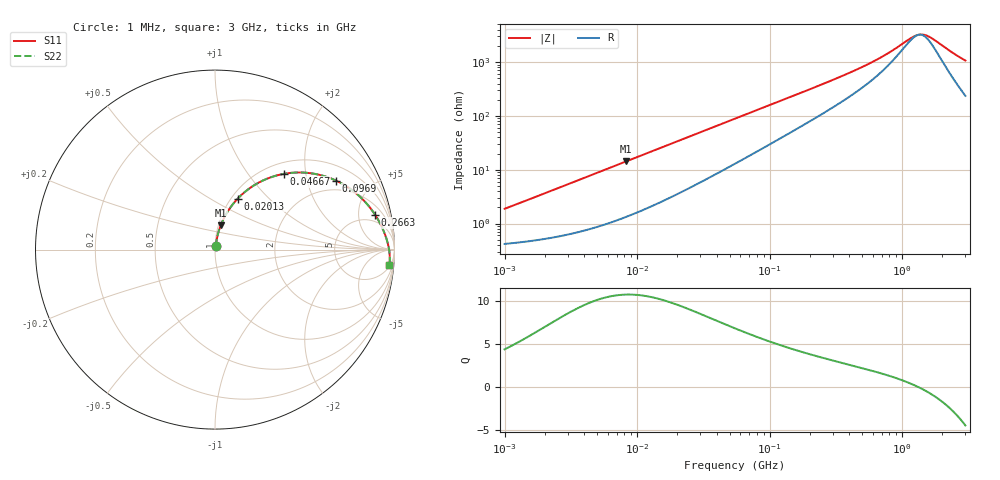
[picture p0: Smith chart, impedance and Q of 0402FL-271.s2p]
# MHz S MA R 50
!Freq  MagS11  AngS11  MagS21  AngS21  MagS12  AngS12  MagS22  AngS22
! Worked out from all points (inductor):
!   801 points, 1 MHz to 3 GHz, reference 50 ohm
!   read as one part in series: L = 289 nH near 1.041 MHz
!   highest Q = 10.7 at 8.262 MHz (marker M1), where L = 274 nH
!   self-resonance near 1.333 GHz
!   S11 on the Smith chart (normalised r, x): 1 MHz: 1.01, +0.04; 20.13 MHz: 1.07, +0.67; 46.67 MHz: 1.21, +1.51; 96.9 MHz: 1.57, +3.03; 266.3 MHz: 3.40, +7.92; 3 GHz: 6, -21
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1  0.0187 76.1  0.9957 -1.0  0.9957 -1.0  0.0187 76.1
3.823119  0.06712 80.1  0.9906 -3.8  0.9906 -3.8  0.06712 80.1
8.262105  0.1396 76.7  0.9773 -8.0  0.9773 -8.0  0.1396 76.7
14.47069  0.2333 71.0  0.95 -13.4  0.95 -13.4  0.2333 71.0
20.13356  0.3106 66.0  0.9187 -18.0  0.9187 -18.0  0.3106 66.0
30.3475  0.4292 58.0  0.8542 -25.2  0.8542 -25.2  0.4292 58.0
46.66789  0.5693 47.8  0.748 -34.3  0.748 -34.3  0.5693 47.8
54.77226  0.6208 43.7  0.6989 -37.9  0.6989 -37.9  0.6208 43.7
71.76513  0.7012 36.9  0.6084 -43.8  0.6084 -43.8  0.7012 36.9
96.89593  0.776 29.7  0.5041 -49.7  0.5041 -49.7  0.776 29.7
140.3209  0.8446 22.0  0.3835 -55.6  0.3835 -55.6  0.8446 22.0
209.4008  0.8933 15.4  0.2743 -59.6  0.2743 -59.6  0.8933 15.4
266.2515  0.9134 12.2  0.2208 -60.9  0.2208 -60.9  0.9134 12.2
500.1674  0.9462 6.1  0.1165 -59.5  0.1165 -59.5  0.9462 6.1
792.5923  0.96 3.0  0.06455 -50.2  0.06455 -50.2  0.96 3.0
1206.698  0.9684 0.6  0.03301 -16.4  0.03301 -16.4  0.9684 0.6
1320.433  0.9698 0.1  0.03024 -1.7  0.03024 -1.7  0.9698 0.1
1430.499  0.9709 -0.4  0.02988 12.9  0.02988 12.9  0.9709 -0.4
1534.307  0.9718 -0.8  0.03129 25.3  0.03129 25.3  0.9718 -0.8
1662.201  0.9728 -1.2  0.03468 37.6  0.03468 37.6  0.9728 -1.2
2431.346  0.9756 -3.6  0.06669 66.8  0.06669 66.8  0.9756 -3.6
3000  0.9758 -5.1  0.09138 72.1  0.09138 72.1  0.9758 -5.1
